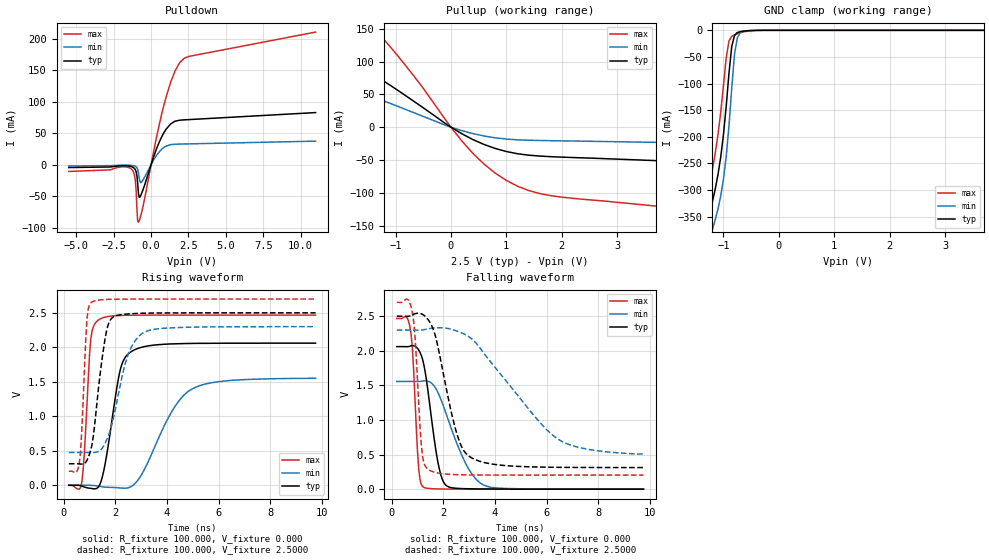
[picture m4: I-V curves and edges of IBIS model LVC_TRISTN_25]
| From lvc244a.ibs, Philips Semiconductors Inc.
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|   Model LVC_TRISTN_25
[Model]   LVC_TRISTN_25
Model_type   3-state
Polarity   Non-Inverting
Enable   Active-Low
Vmeas =  1.25000V
Cref  = 50.0000pF
Rref  =  0.5000k
Vref  =  0.000V
C_comp   3.40pF   2.95pF   3.93pF
[Model Spec]
| Note: The input and output voltage ratings may be exceeded if the input and
|   output current ratings are observed (please refer to the data sheet)
|   Subparameter   typ   min   max
| Timing Thresholds
Vmeas   1.25   1.15   1.5
|Ambient temperature:   25.0000   85.0000   -40.0000
[Temperature Range]   35.0000   95.0000   -30.0000
[Voltage Range]   2.5000V   2.3000V   2.7000V
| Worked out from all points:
|   slope of the pulldown table from 0 to 0.375 V, typ, clamps not added: 14.5 ohm
|   slope of the pullup table from 0 to 0.375 V, typ, clamps not added: 20.9 ohm
|   GND clamp passes 1 mA (typ) near -0.58 V on its own axis
|   rising waveform, R_fixture 100.000, V_fixture 0.000: 20-80 % time 523ps typ, 1.27ns min, 214ps max; typ from 0 V to 2.06 V
|   rising waveform, R_fixture 100.000, V_fixture 2.5000: 20-80 % time 417ps typ, 701ps min, 182ps max; typ from 0.312 V to 2.5 V
|   falling waveform, R_fixture 100.000, V_fixture 0.000: 20-80 % time 463ps typ, 991ps min, 198ps max; typ from 2.06 V to 0 V
|   falling waveform, R_fixture 100.000, V_fixture 2.5000: 20-80 % time 779ps typ, 2.36ns min, 231ps max; typ from 2.5 V to 0.312 V
|Process Range   nominal   slow   fast
[Pulldown]
| voltage   I(typ)   I(min)   I(max)
-5.5V     -4.613mA   -2.143mA   -10.81mA
-1.35V    -2.944mA   -1.155mA   -6.414mA
-1.05V    -8.191mA   -2.697mA   -25.91mA
-900mV    -29.25mA   -7.337mA   -88.93mA
-850mV    -44.66mA   -12.7mA    -91.32mA
-650mV    -46.54mA   -27.94mA   -77.25mA
300mV     21.1mA     12.41mA    36.29mA
900mV     52.38mA    27.94mA    98.2mA
1.3V      64.49mA    31.72mA    130.2mA
1.9V      70.44mA    32.61mA    161.5mA
2.5V      71.41mA    32.93mA    171.6mA
11V       82.58mA    37.26mA    210.3mA
[Pullup]
| voltage   I(typ)   I(min)   I(max)
-8.7V     182.7mA    80.27mA    555.2mA
-2.9V     153.2mA    80.27mA    293.7mA
-2.3V     126.7mA    71.11mA    239.9mA
-1.5V     85.64mA    49.05mA    161.6mA
-1.3V     74.96mA    42.81mA    142.4mA
-1.1V     64.03mA    36.38mA    122.9mA
400mV     -19.05mA   -9.895mA   -40.21mA
800mV     -32.49mA   -16.27mA   -70.04mA
1.4V      -42.71mA   -19.95mA   -96.54mA
2.2V      -46.34mA   -21.15mA   -108.5mA
7.6V      -63.68mA   -28.65mA   -152.4mA
8.2V      -65.63mA   -29.49mA   -157.3mA
[GND_clamp]
| voltage   I(typ)   I(min)   I(max)
-5.5V     -4.538A    -4.57A     -4.506A
-1.35V    -431mA     -477.3mA   -376.9mA
-1.3V     -386.8mA   -433.7mA   -332mA
-1.2V     -322.6mA   -374.6mA   -261.8mA
-1.05V    -238.7mA   -311.7mA   -154.9mA
-950mV    -142.7mA   -237.3mA   -51.59mA
-900mV    -80.46mA   -179.9mA   -19.99mA
-850mV    -30.44mA   -108.2mA   -11.38mA
-800mV    -9.76mA    -44.83mA   -8.484mA
-750mV    -4.198mA   -14.39mA   -6.448mA
-700mV    -2.54mA    -4.591mA   -4.706mA
5.5V      588.5pA    6.601nA    16.7pA
[Ramp]
| variable   typ   min   max
dV/dt_r   1.236V/522.731ps   931.056mV/1.268ns   1.480V/214.373ps
dV/dt_f   1.313V/779.404ps   1.077V/2.370ns   1.498V/230.443ps
R_load = 100.000
[Rising Waveform]
R_fixture   = 100.000
V_fixture   = 0.000
V_fixture_min = 0.000
V_fixture_max = 0.000
| time   V(typ)   V(min)   V(max)
200ps     -44.23uV   -9.382uV   -62.91uV
700ps     -11.68mV   354.8uV    39.79mV
800ps     -24.48mV   739.8uV    473.9mV
1.05ns    -45.18mV   -397.6uV   2.124V
1.35ns    -22.07mV   -13.23mV   2.398V
1.6ns     302.7mV    -26.86mV   2.438V
2.2ns     1.689V     -39.02mV   2.462V
2.6ns     1.934V     -20.67mV   2.465V
5ns       2.057V     1.403V     2.467V
9.75ns    2.061V     1.551V     2.467V
[Rising Waveform]
R_fixture   = 100.000
V_fixture   = 2.5000
V_fixture_min = 2.3000
V_fixture_max = 2.7000
| time   V(typ)   V(min)   V(max)
200ps     312.1mV    475.7mV    203.5mV
600ps     310.1mV    475.9mV    307mV
700ps     307.2mV    476.2mV    792.3mV
900ps     360.7mV    475.9mV    2.407V
1.1ns     596.5mV    473.9mV    2.659V
1.6ns     2.121V     609.4mV    2.693V
1.9ns     2.436V     935.8mV    2.697V
2.5ns     2.484V     1.902V     2.7V
3.2ns     2.495V     2.233V     2.7V
9.75ns    2.5V       2.3V       2.7V
[Falling Waveform]
R_fixture   = 100.000
V_fixture   = 0.000
V_fixture_min = 0.000
V_fixture_max = 0.000
| time   V(typ)   V(min)   V(max)
200ps     2.061V     1.557V     2.467V
600ps     2.059V     1.557V     2.477V
750ps     2.072V     1.557V     2.249V
1.05ns    2.011V     1.557V     286.5mV
1.25ns    1.795V     1.565V     25.54mV
1.8ns     375.5mV    1.392V     3.701mV
2.15ns    43.12mV    1.048V     1.77mV
2.95ns    5.87mV     313.2mV    364.1uV
3.6ns     2.785mV    53.06mV    97.35uV
9.75ns    1.767uV    450.5uV    -471pV
[Falling Waveform]
R_fixture   = 100.000
V_fixture   = 2.5000
V_fixture_min = 2.3000
V_fixture_max = 2.7000
| time   V(typ)   V(min)   V(max)
200ps     2.5V       2.3V       2.7V
800ps     2.52V      2.3V       2.56V
900ps     2.535V     2.299V     2.242V
1.15ns    2.535V     2.299V     636.7mV
1.45ns    2.431V     2.321V     278mV
1.7ns     2.208V     2.331V     240.9mV
2.5ns     833.6mV    2.289V     210.1mV
3ns       476.2mV    2.201V     206mV
6.5ns     315.6mV    708.8mV    203.6mV
9.75ns    312.3mV    508.5mV    203.5mV
